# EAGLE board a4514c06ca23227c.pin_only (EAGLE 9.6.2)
REV: B

Size 30.35 x 12.06 mm. Coordinates in mm from the lower left corner, seen from the top.
Outline: 0,10.79 arc-90 1.33,12.06 29.15,12.06 arc-90 30.35,10.79 30.35,1.27 arc-90 29.08,0 1.27,0 arc-90 0,1.27 0,10.79
Copper layers (1*16): Top 0.035mm / dielectric 1.5mm / Bottom 0.035mm
Design rules "adafruit": minimum track width 8mil, minimum drill 16mil, track to track 8mil, track to pad 8mil, pad to pad 8mil, via to via 8mil, smd to smd 8mil, copper to edge 10mil, drill to drill 8mil, minimum pad ring 10mil, minimum via ring 8mil, stop-mask expansion 4mil, vias tented up to drill 20mil, thermal gap 10mil

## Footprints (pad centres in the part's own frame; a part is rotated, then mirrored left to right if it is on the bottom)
0805-NO = smd 1.24 x 1.5: 1 -0.95,0; 2 0.95,0
FIDUCIAL_1MM = smd 1 x 1: 1 0,0
CHIPLED_0603_NOOUTLINE = smd 0.8 x 0.8: A 0,-0.75; C 0,0.75
0603-NO = smd 1.075 x 1: 1 -0.85,0; 2 0.85,0
EG1390 = smd 1 x 1.5: O1 -2.5,2.8; O2 -2.5,-2.8; P1 0,2.8; P2 0,-2.8; S1 2.5,2.8; S2 2.5,-2.8 | hole 1: 1.5,0; -1.5,0
SOT23-5 = smd 0.55 x 1.2: 1 -0.95,-1.3; 2 0,-1.3; 3 0.95,-1.3; 4 0.95,1.3; 5 -0.95,1.3
USBA_PCB = smd 7.5 x 1.5: GND -0.2,3.5; VCC -0.2,-3.5 | smd 6.5 x 1: USB_NEG 0.3,-1; USB_PLUS 0.3,1
JSTPH2_BATT = smd 1 x 4.6: 1 -1,-2.049; 2 1,-2.049 | smd 1.6 x 3.4: NC1 -3.4,3.151; NC2 3.4,3.151

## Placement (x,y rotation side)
C1  10uF  [0805-NO]  12.06,7.75 270 top
C2  10uF  [0805-NO]  21.21,9.72 270 top
FID1  FIDUCIAL_1MM  [FIDUCIAL_1MM]  27.5,6.03 0 top
LED1  RED  [CHIPLED_0603_NOOUTLINE]  11.81,10.16 270 top
LED2  GREEN  [CHIPLED_0603_NOOUTLINE]  12,1.84 270 top
PLABEL0  [PLABEL0]  9.78,10.79 0 top
PLABEL1  [PLABEL1]  9.21,0.19 0 top
PLABEL2  [PLABEL2]  22.61,10.67 0 top
PLABEL3  [PLABEL3]  23.75,0.38 0 top
PLABEL4  [PLABEL4]  15.18,0.95 0 top
PLABEL5  [PLABEL5]  17.53,1.02 0 top
PLABEL6  [PLABEL6]  12.95,2.86 90 top
PLABEL7  [PLABEL7]  17.65,6.67 0 top
PLABEL8  [PLABEL8]  15.11,6.67 0 top
PLABEL9  [PLABEL9]  23.24,4.95 0 bottom
PLABEL10  [PLABEL10]  4,6.1 90 bottom
PLABEL11  [PLABEL11]  24.51,10.29 0 bottom
R1  2K  [0603-NO]  13.78,9.65 270 top
R2  10K  [0603-NO]  11.3,4.38 90 top
R3  10K  [0603-NO]  15.11,9.65 90 top
R4  2K  [0603-NO]  21.27,1.97 270 top
SW1  DPDT Switch  [EG1390]  16.76,4.38 180 top
U1  MCP73831T-2ACI/OT  [SOT23-5]  17.91,9.78 90 top
U$8  [ADAFRUIT_TEXT_20MM]  29.72,0.13 0 bottom
U$9  [PCBFEAT-REV-040]  28.07,10.6 0 bottom
X1  PCBUSB  [USBA_PCB]  4.95,6.03 0 top
X3  CON_JST_PH_2PIN_MT_BATT  [JSTPH2_BATT]  25.08,6.03 270 top

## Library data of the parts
C1 C2 R1-R3 U$8 = microbuilder
FID1 = microbuilder; BOM: EXCLUDE
LED1 LED2 = microbuilder; JLC_ROTATION: 270
PLABEL0 PLABEL1-PLABEL11 = pinguin
R4 = microbuilder; AUTHOR: K. TOWNSEND
SW1 = adafruit_electromech; LCSC: C2837066
U1 = microbuilder; JLC_ROTATION: 270; LCSC: C424093
U$9 = microbuilder; REV: B
X1 = adafruit_electromech
X3 = adafruit_electromech; LCSC: C47647

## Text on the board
Pinguin_tBackup: CHG | MicroLipo | 1 | 5 | Rate | L | H | DONE | 3.7/4.2V
Pinguin_bBackup: Adafruit MicroLipo | Plug into USB | 3.7V/4.2V LiPoly/LiIon / 100mA/500mA Rate / Battery Charger

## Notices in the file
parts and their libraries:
microbuilder: This work is placed in the public domain, and may be freely used for commercial and non-commercial work with the following conditions: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
